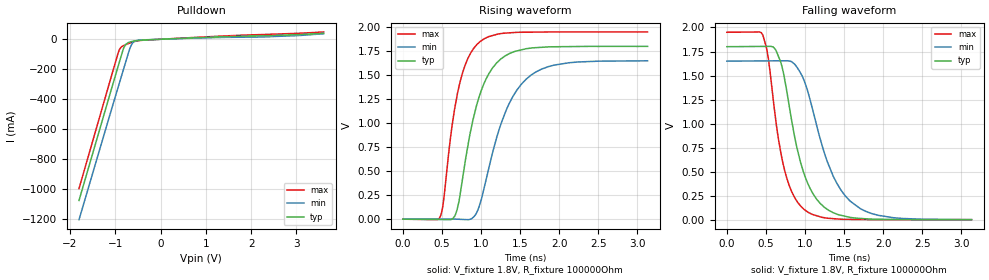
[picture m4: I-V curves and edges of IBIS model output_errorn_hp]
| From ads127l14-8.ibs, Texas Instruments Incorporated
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|   output_errorn_hp Model
[Model]   output_errorn_hp
Model_type   Open_drain
Polarity   Non-Inverting
Vmeas = 0.9
Vref = 1.8
Cref = 2pF
Rref = 100000
|   typ   min   max
C_comp   0.591pF   0.619pF   0.582pF
[Voltage Range]   1.8   1.65   1.95
[Temperature Range]   27   125   -40
[Pullup Reference]   1.8   1.65   1.95
[Pulldown Reference]   0   0   0
[Power Clamp Reference]   1.8   1.65   1.95
[GND Clamp Reference]   0   0   0
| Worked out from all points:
|   slope of the pulldown table from 0 to 0.27 V, typ, clamps not added: 75 ohm
|   falling waveform, V_fixture 1.8V, R_fixture 100000Ohm: 20-80 % time 301ps typ, 403ps min, 234ps max; typ from 1.8 V to 0.003 V
|   rising waveform, V_fixture 1.8V, R_fixture 100000Ohm: 20-80 % time 301ps typ, 398ps min, 230ps max; typ from 0.003 V to 1.8 V
[Pulldown]
|   Voltage   I(typ)   I(min)   I(max)
-1.8V     -1.076A    -1.205A    -996.8mA
-1.071V   -318.7mA   -456.5mA   -231.6mA
-914.4mV  -157.8mA   -298mA     -73.35mA
-871.2mV  -113.9mA   -254.4mA   -52.72mA
-817.2mV  -61.32mA   -199.9mA   -42.37mA
-774mV    -36.03mA   -156.4mA   -36.65mA
-671.4mV  -17.84mA   -56.07mA   -24.27mA
-639mV    -15.21mA   -34.51mA   -20.79mA
-590.4mV  -11.97mA   -16.66mA   -16.19mA
-369mV    -5.011mA   -4.066mA   -6.238mA
2.261V    22.91mA    15.46mA    31.55mA
3.6V      39.89mA    36.84mA    48.71mA
[Ramp]
R_load = 100000
|   typ   min   max
dV/dt_r   1.07841/3.0082e-10   0.9883/3.9754e-10   1.16849/2.30471e-10
dV/dt_f   1.07841/3.00388e-10   0.9883/4.02538e-10   1.16849/2.34111e-10
[Falling Waveform]
V_fixture = 1.8V
V_fixture_min = 1.65V
V_fixture_max = 1.95V
R_fixture = 100000Ohm
C_fixture = 0F
|   Time   V(typ)   V(min)   V(max)
0s        1.8V       1.65V      1.95V
458.5ps   1.803V     1.652V     1.923V
527.4ps   1.803V     1.653V     1.696V
620.2ps   1.773V     1.653V     1.073V
718.5ps   1.547V     1.654V     586mV
991.8ps   471.4mV    1.442V     106.8mV
1.288ns   108.6mV    600.1mV    17.74mV
1.577ns   26.17mV    196mV      5.616mV
2.13ns    4.778mV    22.93mV    2.437mV
3.13ns    2.647mV    2.823mV    2.437mV
[Rising Waveform]
V_fixture = 1.8V
V_fixture_min = 1.65V
V_fixture_max = 1.95V
R_fixture = 100000Ohm
C_fixture = 0F
|   Time   V(typ)   V(min)   V(max)
0s        2.653mV    2.831mV    2.512mV
476.6ps   -973.2uV   3.108mV    26.61mV
637.4ps   7.566mV    3.201mV    1.023V
718.5ps   196.2mV    1.741mV    1.388V
860ps     896.7mV    2.048mV    1.721V
991.8ps   1.317V     178.8mV    1.853V
1.257ns   1.672V     1V         1.933V
1.577ns   1.776V     1.459V     1.948V
2.13ns    1.798V     1.63V      1.95V
3.13ns    1.8V       1.65V      1.95V
